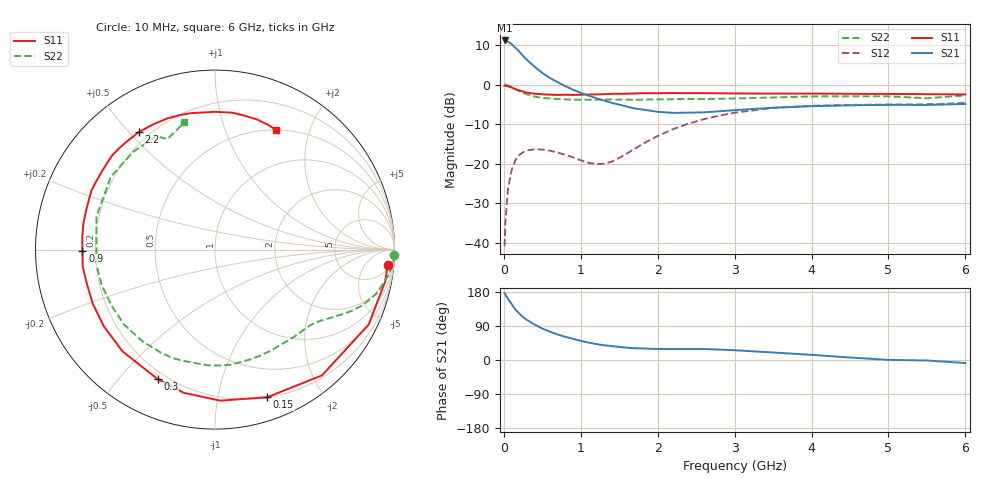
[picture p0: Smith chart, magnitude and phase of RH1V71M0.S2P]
! SIEMENS Small Signal Semiconductors
! BFR106
! Si NPN RF Bipolar Junction Transistor in SOT23
! VCE = 1.75 V  IC = 1 mA
! Common Emitter S-Parameters:  August  1996
# GHz  S  MA  R  50
!  f  S11  S21  S12  S22
! GHz  MAG  ANG  MAG  ANG  MAG  ANG  MAG  ANG
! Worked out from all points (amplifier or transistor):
!   36 points, 10 MHz to 6 GHz, reference 50 ohm
!   highest |S21| = 11.2 dB at 10 MHz (marker M1)
!   |S21| within 3 dB of that: start of sweep to 208.3 MHz
!   unconditionally stable (mu >= 1): 856.3 MHz to end of sweep
!   at 250 MHz: K = 0.27, MSG = 12.2 dB, |S12| = -17.1 dB
!   at 1.4 GHz: K = 1.51, MAG = 3.2 dB, |S12| = -19.5 dB
!   at 6 GHz: K = 1.02, MAG = -1.0 dB, |S12| = -4.7 dB
!   S11 on the Smith chart (normalised r, x): 10 MHz: 7, -19; 150 MHz: 0.20, -1.40; 300 MHz: 0.17, -0.64; 900 MHz: 0.15, -0.01; 2.2 GHz: 0.16, +0.53; 6 GHz: 0.50, +1.51
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0.01  0.966 -5.2  3.615 175.9  0.009 88.3  0.9999 -1.8
0.02  0.9646 -10.7  3.612 173.2  0.018 82.0  0.9991 -3.4
0.05  0.9527 -26.0  3.51 162.4  0.0446 74.4  0.9785 -8.2
0.1  0.92 -49.6  3.249 147.8  0.0825 62.2  0.9335 -15.2
0.15  0.8726 -70.5  2.918 133.4  0.11 50.1  0.8779 -20.8
0.2  0.842 -88.0  2.612 122.8  0.128 41.9  0.828 -24.6
0.25  0.8168 -102.3  2.309 113.1  0.1397 34.5  0.7823 -27.9
0.3  0.7891 -113.9  2.055 105.7  0.1464 29.3  0.752 -30.2
0.4  0.7661 -132.3  1.682 93.4  0.1517 21.1  0.705 -34.4
0.5  0.7524 -145.5  1.399 83.0  0.1503 15.6  0.6782 -38.4
0.7  0.7389 -165.3  1.071 67.4  0.1375 10.6  0.6569 -47.2
0.9  0.7386 -179.3  0.86 55.7  0.1195 12.0  0.6437 -56.4
1.1  0.7474 168.7  0.724 46.0  0.1022 21.0  0.6428 -66.8
1.4  0.7632 154.4  0.587 36.7  0.1055 47.5  0.6472 -82.7
1.9  0.7772 133.7  0.467 29.5  0.1993 66.0  0.6489 -111.1
2.2  0.7803 123.0  0.438 29.0  0.2725 63.0  0.6515 -128.3
2.8  0.7748 104.7  0.459 27.5  0.4039 48.9  0.6615 -162.5
3.5  0.7676 90.1  0.509 19.8  0.5053 31.3  0.6856 164.5
4.5  0.7636 76.6  0.546 6.6  0.5521 11.0  0.7105 129.7
5  0.7615 71.7  0.553 0.3  0.5581 3.6  0.7101 117.4
5.5  0.755 66.7  0.552 -1.3  0.5624 0.3  0.6712 113.2
6  0.7491 63.2  0.568 -8.0  0.5836 -7.1  0.7288 103.5
